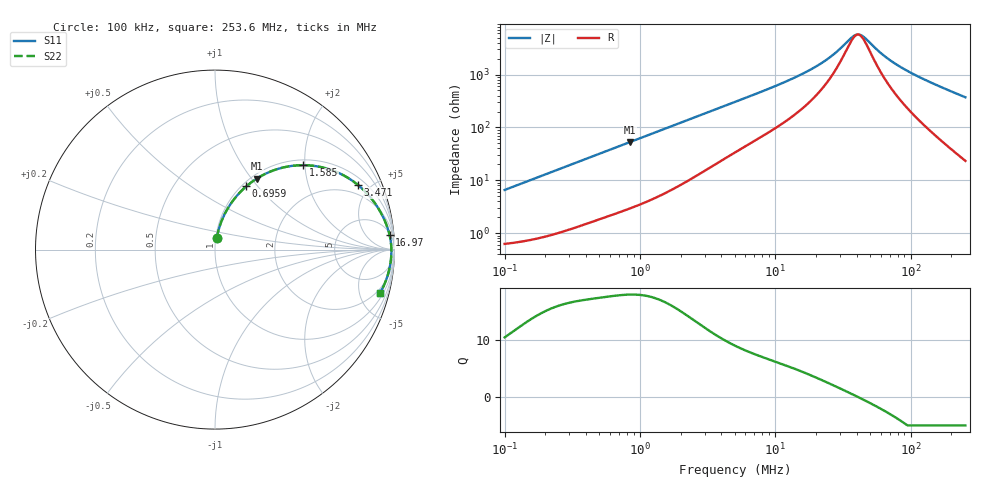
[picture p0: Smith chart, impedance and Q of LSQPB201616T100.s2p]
! LSQPB201616T100  S-PARAMETER MODEL  ( General Type )
! Model Generated by TAIYO YUDEN Corporation (http://www.ty-top.com)
! Version 2.0
! TAIYO YUDEN Control No. 100810NC14SB-FKC
! Copyright(c) 2008 TAIYO YUDEN CO.,LTD. All Rights Reserved.
! Product Description (link to TY-COMPAS)
! https://ds.yuden.co.jp/TYCOMPAS/or/detail?pn=LSQPB201616T100K&u=M
! Products Name : Inductors
! Characteristics :
!  Inductance : 10 uH , SRF(min) : 35 MHz , DC Resistance(max) : 0.52 Ohm
!  Rated Current : Saturation :450 mA , Temp Rise : 520 mA (40 degC)
!  Case Size : 2.0 x 1.6 / 0.079 x 0.063 [mm/inch] , Thickness : 1.6 / 0.063 [mm/inch]
!  (Conditions: Temperature = 25 degC , DC Bias Current/Voltage = 0A / 0V)
! External Node Assignments :
!  1  o---GGG---o  2
! GND o---------o GND
! Frequency Range : 0.1MHz  -  253.640152MHz  [ 402 STEP ]
# MHz S RI R 50
! Freq[MHz].  S11 Real  S11 Imag  S21 Real  S21 Imag  S12 Real  S12 Imag  S22 Real  S22 Imag
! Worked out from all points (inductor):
!   401 points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, 100 kHz to 253.6 MHz, reference 50 ohm
!   read as one part in series: L = 10.4 uH near 104 kHz
!   highest Q = 17.9 at 846.5 kHz (marker M1), where L = 9.95 uH
!   self-resonance near 40.71 MHz
!   S11 on the Smith chart (normalised r, x): 100 kHz: 1.01, +0.13; 695.9 kHz: 1.05, +0.87; 1.585 MHz: 1.12, +1.96; 3.471 MHz: 1.38, +4.21; 16.97 MHz: 6, +22; 253.6 MHz: 1.47, -7.42
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0.1  0.0104 0.0644  0.9896 -0.0644  0.9896 -0.0644  0.0104 0.0644
0.19855  0.0244 0.1245  0.9756 -0.1245  0.9756 -0.1245  0.0244 0.1245
0.371712  0.0652 0.2191  0.9348 -0.2191  0.9348 -0.2191  0.0652 0.2191
0.695895  0.1743 0.3524  0.8257 -0.3524  0.8257 -0.3524  0.1743 0.3524
0.846544  0.2317 0.395  0.7683 -0.395  0.7683 -0.395  0.2317 0.395
1.381698  0.4276 0.4663  0.5724 -0.4663  0.5724 -0.4663  0.4276 0.4663
1.584845  0.4908 0.4704  0.5092 -0.4704  0.5092 -0.4704  0.4908 0.4704
2.255156  0.6481 0.4436  0.3519 -0.4436  0.3519 -0.4436  0.6481 0.4436
3.470633  0.7968 0.36  0.2032 -0.36  0.2032 -0.36  0.7968 0.36
5.03627  0.8775 0.2768  0.1225 -0.2768  0.1225 -0.2768  0.8775 0.2768
10.19738  0.9515 0.1479  0.0485 -0.1479  0.0485 -0.1479  0.9515 0.1479
16.97316  0.9725 0.0821  0.0275 -0.0821  0.0275 -0.0821  0.9725 0.0821
18.72042  0.9749 0.0715  0.0251 -0.0715  0.0251 -0.0715  0.9749 0.0715
25.6144  0.98 0.0405  0.02 -0.0405  0.02 -0.0405  0.98 0.0405
36.44803  0.9825 0.00943  0.0175 -0.00943  0.0175 -0.00943  0.9825 0.00943
40.20007  0.9828 0.00108  0.0172 -0.00108  0.0172 -0.00108  0.9828 0.00108
45.21578  0.9829 -0.00896  0.0171 0.00896  0.0171 0.00896  0.9829 -0.00896
58.33472  0.9823 -0.0314  0.0177 0.0314  0.0177 0.0314  0.9823 -0.0314
69.58603  0.981 -0.0479  0.019 0.0479  0.019 0.0479  0.981 -0.0479
88.03362  0.9781 -0.0723  0.0219 0.0723  0.0219 0.0723  0.9781 -0.0723
118.1155  0.9715 -0.108  0.0285 0.108  0.0285 0.108  0.9715 -0.108
253.6402  0.9193 -0.2428  0.0807 0.2428  0.0807 0.2428  0.9193 -0.2428
